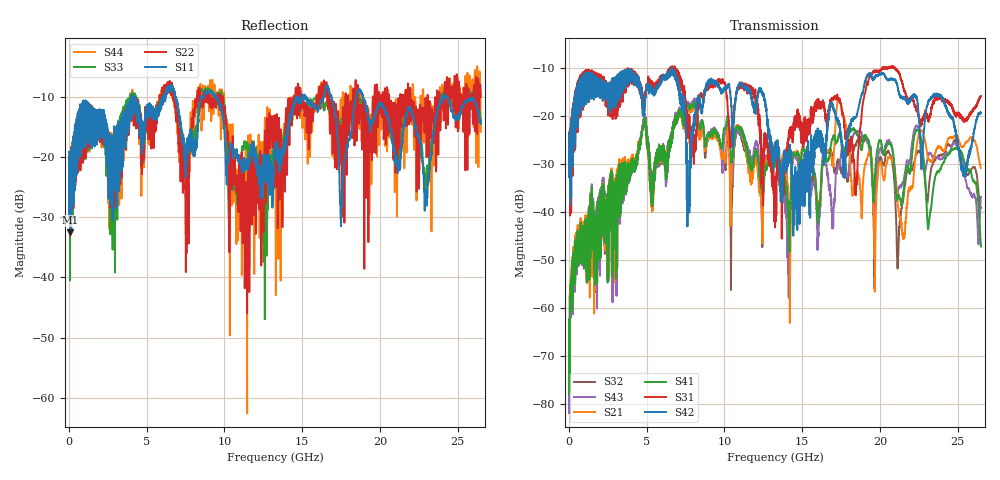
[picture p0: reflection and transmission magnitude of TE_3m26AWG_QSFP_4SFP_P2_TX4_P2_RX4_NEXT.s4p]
!Agilent Technologies,N5222A,MY51421691,A.10.00.00
!Agilent N5222A: A.10.00.00
!Date: Friday, January 30, 2015 12:36:19
!Correction: S11(Full 4 Port(1,2,3,4))
!S12(Full 4 Port(1,2,3,4))
!S13(Full 4 Port(1,2,3,4))
!S14(Full 4 Port(1,2,3,4))
!S21(Full 4 Port(1,2,3,4))
!S22(Full 4 Port(1,2,3,4))
!S23(Full 4 Port(1,2,3,4))
!S24(Full 4 Port(1,2,3,4))
!S31(Full 4 Port(1,2,3,4))
!S32(Full 4 Port(1,2,3,4))
!S33(Full 4 Port(1,2,3,4))
!S34(Full 4 Port(1,2,3,4))
!S41(Full 4 Port(1,2,3,4))
!S42(Full 4 Port(1,2,3,4))
!S43(Full 4 Port(1,2,3,4))
!S44(Full 4 Port(1,2,3,4))
!S4P File: Measurements: <S11,S12,S13,S14>,
!<S21,S22,S23,S24>,
!<S31,S32,S33,S34>,
!<S41,S42,S43,S44>:
# Hz S  dB  R 50.0
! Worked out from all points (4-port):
!   2650 points, 10 MHz to 26.5 GHz, reference 50 ohm
!   strongest paths, dB at 10 MHz, 6.63 GHz, 13.26 GHz, 19.88 GHz, 26.5 GHz:
!     S42: -25.0, -11.1, -25.5, -11.3, -19.3
!     S31: -25.0, -10.5, -43.2, -10.4, -15.7
!     S41: -78.0, -23.2, -29.7, -26.2, -47.2
!     S21: -74.3, -23.4, -28.0, -31.5, -30.8
!     S43: -76.7, -22.6, -29.7, -28.7, -36.8
!     S32: -75.4, -22.8, -29.9, -30.8, -39.0
!   lowest |S11| = -32.5 dB at 70 MHz (marker M1), VSWR 1.05, Z = 52.4 + j0.254 ohm
!   |S11| at or under -10 dB: start of sweep to 4.075 GHz; 9.453 GHz to 14.73 GHz (5.275 GHz wide, 43.6 % of centre); 18.91 GHz to 24.14 GHz (5.227 GHz wide, 24.3 % of centre)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
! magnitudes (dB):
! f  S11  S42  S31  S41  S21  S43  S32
! 10 MHz  -19.2  -25.0  -25.0  -78.0  -74.3  -76.7  -75.4
! 70 MHz  -32.5  -38.5  -40.7  -60.7  -59.1  -62.6  -60.7
! 6.66 GHz  -8.7  -11.0  -10.3  -23.3  -23.2  -22.7  -22.6
! 7.6 GHz  -17.0  -29.0  -19.0  -17.4  -18.0  -17.0  -17.6
! 14.1 GHz  -15.1  -28.3  -25.3  -41.0  -36.4  -49.1  -40.9
! 22.42 GHz  -16.2  -17.2  -19.0  -22.9  -25.1  -22.2  -27.4
! 26.5 GHz  -14.1  -19.3  -15.7  -47.2  -30.8  -36.8  -39.0
